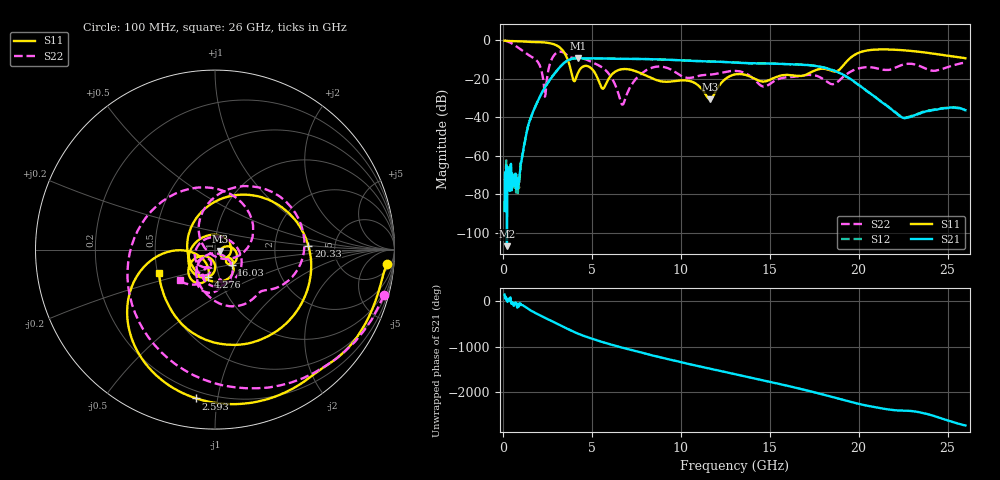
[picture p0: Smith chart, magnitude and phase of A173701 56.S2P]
!  2-Port S-parameters saved by WinCal
! VAR MeasName=S-Parameters (CALIBRATED_DATA) read from VNA (N5245A)
! VAR MeasDate=2017-6-7 10:32:06
! VAR NAME=A173701 56
! VAR FILENAME=A173701 56.S2P
! VAR DATE=2017-6-7 10:32:06
! VAR PHYS_PORTS=1,2
# Hz S DB R 50
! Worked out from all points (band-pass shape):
!   801 points, 100 MHz to 26 GHz, reference 50 ohm
!   highest |S21| = -9.42 dB at 4.212 GHz (marker M1); lowest = -106.8 dB at 229.5 MHz (marker M2)
!   |S21| within 3 dB of the highest: 3.375 GHz to 15.75 GHz (12.38 GHz wide, 129 % of centre); 15.79184 GHz to 15.8211 GHz (29.26 MHz wide, 0.185 % of centre)
!   lowest |S11| = -30.8 dB at 11.66 GHz (marker M3), VSWR 1.06, Z = 52.9 - j0.794 ohm
!   |S11| at or under -10 dB: 3.639 GHz to 19.45 GHz (15.81 GHz wide, 137 % of centre)
!   |S22| runs from -33.5 to -0.2 dB; largest |S21 - S12| = 0.0036
!   S11 on the Smith chart (normalised r, x): 100 MHz: 9, -20; 2.593 GHz: 0.16, -0.87; 4.276 GHz: 0.88, -0.28; 16.03 GHz: 1.19, -0.20; 20.33 GHz: 3.16, +0.18; 26 GHz: 0.51, -0.15
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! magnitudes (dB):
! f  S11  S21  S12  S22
! 100 MHz  -0.3  -88.6  -72.9  -0.2
! 229.5 MHz  -0.5  -106.8  -77.9  -0.6
! 844.6 MHz  -0.6  -74.8  -79.3  -3.8
! 1.492 GHz  -1.0  -42.3  -42.3  -8.0
! 2.366 GHz  -1.3  -24.5  -24.4  -29.3
! 2.593 GHz  -1.6  -21.3  -21.2  -14.2
! 3.111 GHz  -3.2  -15.0  -15.0  -6.2
! 4.212 GHz  -17.3  -9.4  -9.4  -9.2
! 4.276 GHz  -16.1  -9.4  -9.4  -9.2
! 4.438 GHz  -14.2  -9.5  -9.5  -9.4
! 5.636 GHz  -25.2  -9.5  -9.5  -14.6
! 6.737 GHz  -15.1  -9.7  -9.7  -33.4
! 8.744 GHz  -21.1  -10.0  -10.0  -13.7
! 11.66 GHz  -30.8  -11.1  -11.1  -17.9
! 13.05 GHz  -17.8  -11.7  -11.7  -16.0
! 14.67 GHz  -21.5  -12.1  -12.1  -24.1
! 16.03 GHz  -18.1  -12.5  -12.5  -19.2
! 17.39 GHz  -16.4  -13.2  -13.2  -18.1
! 18.55 GHz  -16.2  -15.6  -15.6  -22.9
! 20.33 GHz  -5.7  -25.5  -25.5  -14.1
! 21.69 GHz  -4.9  -34.9  -34.7  -15.5
! 26 GHz  -9.4  -36.4  -36.3  -11.7
